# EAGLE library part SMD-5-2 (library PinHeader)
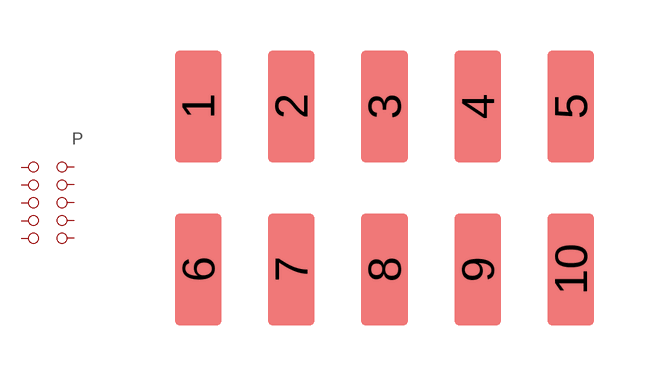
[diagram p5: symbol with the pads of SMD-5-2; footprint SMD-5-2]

Designator prefix P

## SMD-5-2  [SMD-5-2]
1  1  pas
2  2  pas
3  3  pas
4  4  pas
5  5  pas
6  6  pas
7  7  pas
8  8  pas
9  9  pas
10  10  pas

## Footprint SMD-5-2 (pad centres in mm)
smd 1.27 x 3.048: 1 -5.08,2.223; 2 -2.54,2.223; 3 0,2.223; 4 2.54,2.223; 5 5.08,2.223; 6 -5.08,-2.223; 7 -2.54,-2.223; 8 0,-2.223; 9 2.54,-2.223; 10 5.08,-2.223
